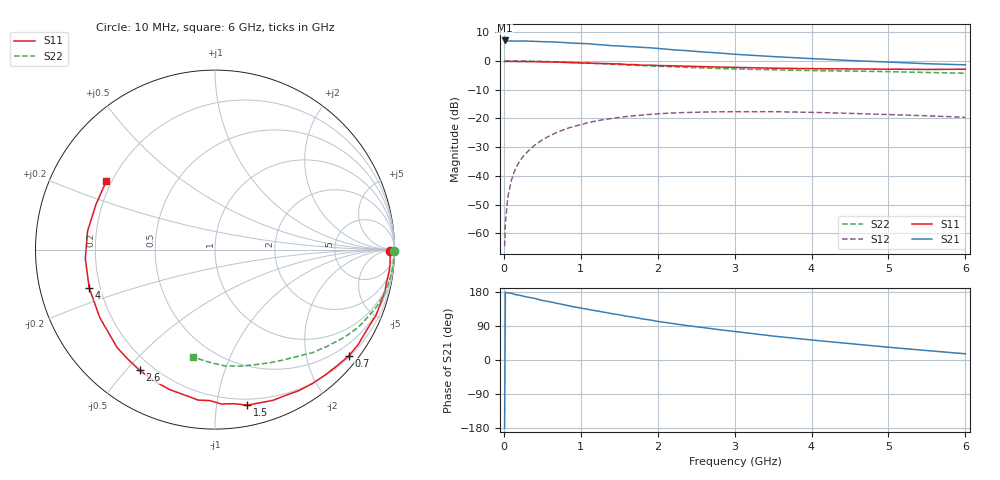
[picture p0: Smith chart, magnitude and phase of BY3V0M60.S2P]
! SIEMENS Small Signal Semiconductors
! BFY420
! Si NPN RF SIEGET Grounded Emitter Transistor in MICRO-X
! VCE = 3 V  IC = 0.6 mA
! Common Emitter S-Parameters:  October  1996
# GHz  S  MA  R  50
!  f  S11  S21  S12  S22
! GHz  MAG  ANG  MAG  ANG  MAG  ANG  MAG  ANG
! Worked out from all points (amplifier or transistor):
!   36 points, 10 MHz to 6 GHz, reference 50 ohm
!   highest |S21| = 7.1 dB at 10 MHz (marker M1)
!   |S21| within 3 dB of that: start of sweep to 2.097 GHz
!   unconditionally stable (mu >= 1): 4.704 GHz to end of sweep
!   at 250 MHz: K = 0.03, MSG = 20.1 dB, |S12| = -33.3 dB
!   at 1.4 GHz: K = 0.17, MSG = 12.7 dB, |S12| = -20.1 dB
!   at 6 GHz: K = 1.41, MAG = 5.3 dB, |S12| = -19.6 dB
!   S11 on the Smith chart (normalised r, x): 10 MHz: 73, -34; 700 MHz: 0.23, -2.85; 1.5 GHz: 0.15, -1.22; 2.6 GHz: 0.15, -0.55; 4 GHz: 0.16, -0.14; 6 GHz: 0.18, +0.28
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0.01  0.9776 -0.6  2.265 -179.3  0.0006 104.8  0.9996 -0.3
0.02  0.9755 -1.2  2.255 178.8  0.0015 90.5  0.9999 -0.6
0.05  0.9771 -2.9  2.214 177.3  0.0042 86.7  0.9991 -1.3
0.1  0.9789 -5.5  2.225 176.0  0.0086 87.9  0.9977 -2.6
0.15  0.9762 -8.4  2.204 172.6  0.0132 84.7  0.9973 -3.9
0.2  0.9725 -11.1  2.213 171.2  0.0176 84.0  0.9965 -5.0
0.25  0.9759 -13.9  2.226 168.7  0.0217 80.8  0.9947 -6.4
0.4  0.9692 -22.2  2.183 162.6  0.0341 76.4  0.9868 -10.2
0.5  0.9568 -27.7  2.158 157.2  0.0423 73.0  0.98 -12.8
0.7  0.9518 -38.5  2.115 149.2  0.0579 66.3  0.9624 -17.7
0.9  0.9294 -49.0  2.037 140.6  0.072 59.4  0.9393 -22.2
1.1  0.9139 -59.4  1.988 133.4  0.0846 53.6  0.916 -26.8
1.5  0.8847 -78.3  1.818 119.4  0.1038 41.8  0.8659 -34.7
1.9  0.8437 -96.4  1.688 105.7  0.1176 32.2  0.8189 -41.8
2.2  0.8199 -108.0  1.558 96.2  0.1243 25.4  0.7907 -46.6
2.6  0.7926 -121.9  1.424 85.4  0.1289 18.2  0.7526 -52.3
2.8  0.7798 -128.7  1.371 80.0  0.1302 14.7  0.7357 -55.3
3.5  0.7454 -149.5  1.188 63.2  0.1308 5.2  0.7001 -64.2
4  0.7323 -163.2  1.095 52.8  0.1274 -0.2  0.6789 -70.8
4.5  0.7242 -176.0  1.014 43.2  0.1223 -4.5  0.6652 -77.5
5.5  0.7093 159.5  0.892 24.9  0.111 -8.5  0.6282 -93.0
6  0.7162 147.7  0.854 16.4  0.1045 -7.9  0.6111 -101.6
